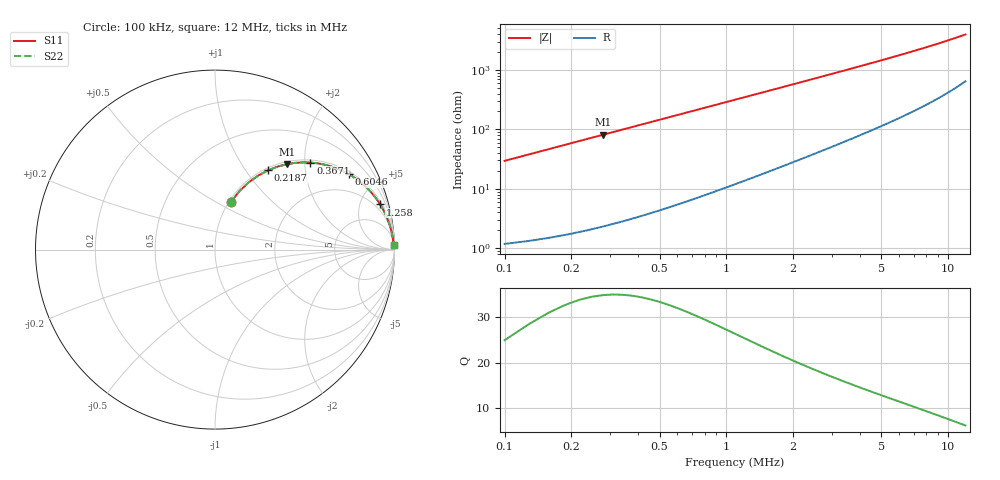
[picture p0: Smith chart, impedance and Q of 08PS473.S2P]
! Coilcraft 0805PS-473 Power Chip Inductor
! 5 February 2003
# MHZ S MA R 50
!Freq  MagS11  AngS11  MagS21  AngS21  MagS12  AngS12  MagS22  AngS22
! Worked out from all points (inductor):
!   402 points, 100 kHz to 12 MHz, reference 50 ohm
!   read as one part in series: L = 46.6 uH near 159.4 kHz
!   highest Q = 34.6 at 278.1 kHz (marker M1), where L = 46.4 uH
!   S11 on the Smith chart (normalised r, x): 100 kHz: 1.02, +0.59; 218.7 kHz: 1.04, +1.28; 367.1 kHz: 1.06, +2.14; 604.6 kHz: 1.11, +3.50; 1.258 MHz: 1.29, +7.22; 12 MHz: 14, +78
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0.1  0.2804 71.4  0.9487 -16.3  0.9487 -16.3  0.2804 71.4
0.15936  0.4189 63.4  0.8947 -24.8  0.8947 -24.8  0.4189 63.4
0.18904  0.4787 59.7  0.8635 -28.6  0.8635 -28.6  0.4787 59.7
0.21872  0.5322 56.2  0.8311 -32.1  0.8311 -32.1  0.5322 56.2
0.27808  0.6216 49.9  0.7658 -38.4  0.7658 -38.4  0.6216 49.9
0.36712  0.7198 42.3  0.6739 -46.0  0.6739 -46.0  0.7198 42.3
0.48584  0.8043 34.8  0.5708 -53.5  0.5708 -53.5  0.8043 34.8
0.60456  0.8567 29.3  0.4898 -58.9  0.4898 -58.9  0.8567 29.3
0.72328  0.8906 25.2  0.4265 -62.9  0.4265 -62.9  0.8906 25.2
0.87168  0.9182 21.4  0.3655 -66.6  0.3655 -66.6  0.9182 21.4
1.04976  0.9389 18.1  0.311 -69.8  0.311 -69.8  0.9389 18.1
1.25752  0.954 15.3  0.2642 -72.4  0.2642 -72.4  0.954 15.3
1.64336  0.9694 11.9  0.2059 -75.6  0.2059 -75.6  0.9694 11.9
2.08856  0.9784 9.4  0.1637 -77.7  0.1637 -77.7  0.9784 9.4
2.50408  0.9831 7.9  0.1372 -79.0  0.1372 -79.0  0.9831 7.9
2.97896  0.9865 6.6  0.1156 -80.0  0.1156 -80.0  0.9865 6.6
4.07712  0.9906 4.8  0.08443 -81.2  0.08443 -81.2  0.9906 4.8
4.9972  0.9923 3.9  0.06853 -81.6  0.06853 -81.6  0.9923 3.9
6.06568  0.9935 3.2  0.05591 -81.8  0.05591 -81.8  0.9935 3.2
8.05424  0.9947 2.3  0.04096 -81.4  0.04096 -81.4  0.9947 2.3
10.0428  0.9953 1.8  0.0316 -80.6  0.0316 -80.6  0.9953 1.8
12  0.9956 1.4  0.02518 -79.2  0.02518 -79.2  0.9956 1.4
